| IBIS file stm32l552_562_wlcsp81_p.ibs
[IBIS ver]   4.2
[File name]  stm32l552_562_wlcsp81_p.ibs
[File Rev]   1.0
[Date]   04-10-2019
[Source]   Data Created at STMicroelectronics
[Notes]   File originated from ELDO simulations.
[Disclaimer] This information is for modeling purpose only and is
   not guaranted.
   The information is subject to change without notice.
[Copyright]  Copyright 2019 STMicroelectronics Inc.
|   Component stm32l552_562_wlcsp81_p
[Component] stm32l552_562_wlcsp81_p
[Manufacturer] STMicroelectronics
[Package]
| variable   typ   min   max
R_pkg  0  NA  NA
L_pkg  0  NA  NA
C_pkg  0  NA  NA
[Pin]   signal_name   model_name R_pin L_pin C_pin
A1 VDD POWER
A2 PC10 io8prog2m25m50m120m_sudq_ft
A3 PD2 io8prog2m25m50m120m_sudq_ft
A4 PG13 io8prog2m25m50m120m_sudq_i2c_ft
A5 VDDIO2 POWER
A6 PB5 io8prog2m25m50m120m_sudq_ft
A7 PB9 io8prog2m25m50m120m_sudq_i2c_ft
A8 VDD12_2 POWER
A9 VDD POWER
B1 VDDUSB POWER
B2 VSS GND
B3 PC12 io8prog2m25m50m120m_sudq_ft
B4 PG12 io8prog2m25m50m120m_sudq_ft
B5 VSS GND
B6 PB4 io8prog2m25m50m120m_sudq_i2c_ft
B7 PC13 io8prog2m25m50m120m_sudq_ft
B8 VSS GND
B9 VBAT POWER
C1 PA11 io8usblsfs_otg2
C2 PA12 io8usblsfs_otg2
C3 PC11 io8prog2m25m50m120m_sudq_ft
C4 PG10 io8prog2m25m50m120m_sudq_ft
C5 PG15 io8prog2m25m50m120m_sudq_ft
C6 PB6 io8prog2m25m50m120m_sudq_i2c_ft
C7 PB8 io8prog2m25m50m120m_sudq_i2c_ft
C8 PC15-OSC32_OUT io8prog2m25m50m120m_sudq_ft
C9 PC14-OSC32_IN io8prog2m25m50m120m_sudq_ft
D1 PA9 io8prog2m25m50m120m_sudq_ft
D2 PA13 io8prog2m25m50m120m_sudq_ft
D3 PA14 io8prog2m25m50m120m_sudq_i2c_ft
D4 PG9 io8prog2m25m50m120m_sudq_ft
D5 PG14 io8prog2m25m50m120m_sudq_i2c_ft
D6 PB7 io8prog2m25m50m120m_sudq_i2c_ft
D7 PH3-BOOT0 io8prog2m25m50m120m_sudq_ft
D8 PH1-OSC_OUT io8prog2m25m50m120m_sudq_ft
D9 PH0-OSC_IN io8prog2m25m50m120m_sudq_ft
E1 PC6 io8prog2m25m50m120m_sudq_ft
E2 PC7 io8prog2m25m50m120m_sudq_ft
E3 PA10 io8prog2m25m50m120m_sudq_ft
E4 PA15 io6usb_bmc_pd_cc_ft
E5 PG11 io8prog2m25m50m120m_sudq_ft
E6 PB3 io8prog2m25m50m120m_sudq_ft
E7 PC0 io8prog2m25m50m120m_sudq_i2c_ft
E8 VSS GND
E9 NRST ioreset_ft_v33
F1 PB15 io6usb_bmc_pd_cc_ft
F2 PB13 io8prog2m25m50m120m_sudq_i2c_ft
F3 PC8 io8prog2m25m50m120m_sudq_ft
F4 PA8 io8prog2m25m50m120m_sudq_i2c_ft
F5 PA3 io8prog2m25m50m120m_sudq_ft
F6 PA1 io8prog2m25m50m120m_sudq_ft
F7 PC2 io8prog2m25m50m120m_sudq_ft
F8 PC1 io8prog2m25m50m120m_sudq_i2c_ft
F9 VDD POWER
G1 PB14 io8prog2m25m50m120m_sudq_i2c_ft
G2 PB12 io8prog2m25m50m120m_sudq_ft
G3 PC9 io8prog2m25m50m120m_sudq_i2c_ft
G4 PC4 io8prog2m25m50m120m_sudq_ft
G5 PA6 io8prog2m25m50m120m_sudq_ft
G6 PA2 io8prog2m25m50m120m_sudq_ft
G7 PC3 io8prog2m25m50m120m_sudq_ft
G8 VREF+ POWER
G9 VSSA_VREF- GND
H1 VDD POWER
H2 VSS GND
H3 PE15 io8prog2m25m50m120m_sudq_ft
H4 PE14 io8prog2m25m50m120m_sudq_ft
H5 PB1 io8prog2m25m50m120m_sudq_ft
H6 PA5 io8prog2m25m50m120m_sudq_ft
H7 PA4 io8prog2m25m50m120m_sudq_ft
H8 PA0 io8prog2m25m50m120m_sudq_ft
H9 VDDA POWER
J1 VDD12_1 POWER
J2 PB11 io8prog2m25m50m120m_sudq_i2c_ft
J3 PB10 io8prog2m25m50m120m_sudq_i2c_ft
J4 PE13 io8prog2m25m50m120m_sudq_ft
J5 PB2 io8prog2m25m50m120m_sudq_ft
J6 PB0 io8prog2m25m50m120m_sudq_ft
J7 PA7 io8prog2m25m50m120m_sudq_i2c_ft
J8 VDD POWER
J9 VSS GND
[Model Selector] io6usb_bmc_pd_cc_ft
usb_bmc_emit_pdccpd  "BMC PD emitter  + PD"
usb_bmc_emit_pdcc3a0  "BMC PD emitter  + 3rd PU"
usb_bmc_emit_pdcc1a5  "BMC PD emitter  + 2nd PU"
usb_bmc_emit_pdccusb  "BMC PD emitter  + 1st PU"
usb_bmc_emit  "BMC PD emitter "
io2_pdcc_ft_3v3_lowspeed  "GPIO-3.3V range - low speed"
io2_pdcc_ft_3v3_mediumspeed  "GPIO-3.3V range - medium speed"
io2_pdcc_ft_3v3_lowspeed_pu  "GPIO-3.3V range - low speed - pull up"
io2_pdcc_ft_3v3_mediumspeed_pu  "GPIO-3.3V range - medium speed - pull up"
io2_pdcc_ft_3v3_lowspeed_pd  "GPIO-3.3V range - low speed - pull down"
io2_pdcc_ft_3v3_mediumspeed_pd  "GPIO-3.3V range - medium speed - pull down"
io2_pdcc_ft_1v8_lowspeed  "GPIO-1.8V range - low speed"
io2_pdcc_ft_1v8_mediumspeed  "GPIO-1.8V range - medium speed"
io2_pdcc_ft_1v8_lowspeed_pu  "GPIO-1.8V range - low speed - pull up"
io2_pdcc_ft_1v8_mediumspeed_pu  "GPIO-1.8V range - medium speed - pull up"
io2_pdcc_ft_1v8_lowspeed_pd  "GPIO-1.8V range - low speed - pull down"
io2_pdcc_ft_1v8_mediumspeed_pd  "GPIO-1.8V range - medium speed - pull down"
io2_pdcc_ft_1v2_lowspeed  "GPIO-1.2V range - low speed"
io2_pdcc_ft_1v2_mediumspeed  "GPIO-1.2V range - medium speed"
io2_pdcc_ft_1v2_lowspeed_pu  "GPIO-1.2V range - low speed - pull up"
io2_pdcc_ft_1v2_mediumspeed_pu  "GPIO-1.2V range - medium speed - pull up"
io2_pdcc_ft_1v2_lowspeed_pd  "GPIO-1.2V range - low speed - pull down"
io2_pdcc_ft_1v2_mediumspeed_pd  "GPIO-1.2V range - medium speed - pull down"
[Model Selector] io8prog2m25m50m120m_sudq_ft
iols8p_sudq_ft_pd_lv  "IO low speed, PD=40kOhm - 1P8V"
iols8p_sudq_ft_pu_lv  "IO low speed, PU=40kOhm - 1P8V"
iols8p_sudq_ft_lv  "IO low speed - 1P8V"
iols8p_sudq_ft_pd  "IO low speed, PD=40kOhm - 3P3V"
iols8p_sudq_ft_pu  "IO low speed, PU=40kOhm - 3P3V"
iols8p_sudq_ft  "IO low speed - 3P3V"
iofs8p_sudq_ft_pd_lv  "IO full speed, PD=40kOhm - 1P8V"
iofs8p_sudq_ft_pu_lv  "IO full speed, PU=40kOhm - 1P8V"
iofs8p_sudq_ft_lv  "IO full speed - 1P8V"
iofs8p_sudq_ft_pd  "IO full speed, PD=40kOhm - 3P3V"
iofs8p_sudq_ft_pu  "IO full speed, PU=40kOhm - 3P3V"
iofs8p_sudq_ft  "IO full speed - 3P3V"
ioms8p_sudq_ft_pd_lv  "IO medium speed, PD=40kOhm - 1P8V"
ioms8p_sudq_ft_pu_lv  "IO medium speed, PU=40kOhm - 1P8V"
ioms8p_sudq_ft_lv  "IO medium speed - 1P8V"
ioms8p_sudq_ft_pd  "IO medium speed, PD=40kOhm - 3P3V"
ioms8p_sudq_ft_pu  "IO medium speed, PU=40kOhm - 3P3V"
ioms8p_sudq_ft  "IO medium speed - 3P3V"
iohs8p_sudq_ft_pd_lv  "IO high speed, PD=40kOhm - 1P8V"
iohs8p_sudq_ft_pu_lv  "IO high speed, PU=40kOhm - 1P8V"
iohs8p_sudq_ft_lv  "IO high speed - 1P8V"
iohs8p_sudq_ft_pd  "IO high speed, PD=40kOhm - 3P3V"
iohs8p_sudq_ft_pu  "IO high speed, PU=40kOhm - 3P3V"
iohs8p_sudq_ft  "IO high speed - 3P3V"
[Model Selector] io8prog2m25m50m120m_sudq_i2c_ft
io8prog_1v8_i2c_pd  "5V Tol GPIO 1.8V range i2c functionality with pull down"
io8prog_1v8_i2c_pu  "5V Tol GPIO 1.8V range i2c functionality with pull up"
io8prog_1v8_i2c  "5V Tol GPIO 1.8V range i2c functionality"
io8prog_3v3_i2c_pd  "5V Tol GPIO 3.3V range i2c functionality with pull down"
io8prog_3v3_i2c_pu  "5V Tol GPIO 3.3V range i2c functionality with pull up"
io8prog_3v3_i2c  "5V Tol GPIO 3.3V range i2c functionality"
iols8p_sudq_ft_pd_lv  "IO low speed, PD=40kOhm - 1P8V"
iols8p_sudq_ft_pu_lv  "IO low speed, PU=40kOhm - 1P8V"
iols8p_sudq_ft_lv  "IO low speed - 1P8V"
iols8p_sudq_ft_pd  "IO low speed, PD=40kOhm - 3P3V"
iols8p_sudq_ft_pu  "IO low speed, PU=40kOhm - 3P3V"
iols8p_sudq_ft  "IO low speed - 3P3V"
iofs8p_sudq_ft_pd_lv  "IO full speed, PD=40kOhm - 1P8V"
iofs8p_sudq_ft_pu_lv  "IO full speed, PU=40kOhm - 1P8V"
iofs8p_sudq_ft_lv  "IO full speed - 1P8V"
iofs8p_sudq_ft_pd  "IO full speed, PD=40kOhm - 3P3V"
iofs8p_sudq_ft_pu  "IO full speed, PU=40kOhm - 3P3V"
iofs8p_sudq_ft  "IO full speed - 3P3V"
ioms8p_sudq_ft_pd_lv  "IO medium speed, PD=40kOhm - 1P8V"
ioms8p_sudq_ft_pu_lv  "IO medium speed, PU=40kOhm - 1P8V"
ioms8p_sudq_ft_lv  "IO medium speed - 1P8V"
ioms8p_sudq_ft_pd  "IO medium speed, PD=40kOhm - 3P3V"
ioms8p_sudq_ft_pu  "IO medium speed, PU=40kOhm - 3P3V"
ioms8p_sudq_ft  "IO medium speed - 3P3V"
iohs8p_sudq_ft_pd_lv  "IO high speed, PD=40kOhm - 1P8V"
iohs8p_sudq_ft_pu_lv  "IO high speed, PU=40kOhm - 1P8V"
iohs8p_sudq_ft_lv  "IO high speed - 1P8V"
iohs8p_sudq_ft_pd  "IO high speed, PD=40kOhm - 3P3V"
iohs8p_sudq_ft_pu  "IO high speed, PU=40kOhm - 3P3V"
iohs8p_sudq_ft  "IO high speed - 3P3V"
[Model Selector] io8usblsfs_otg2
usb_ls_pd  "USB Low Speed mode - Pull Down"
usb_ls_pu2  "USB Low Speed mode - Pull up 2"
usb_ls_pu  "USB Low Speed mode - Pull up"
usb_fs  "USB Low Speed mode"
usb_fs_pd  "USB Full Speed mode - Pull Down"
usb_fs_pu2  "USB Full Speed mode - Pull up 2"
usb_fs_pu  "USB Full Speed mode - Pull up"
[Model Selector] ioreset_ft_v33
ioreset_1v2_pu  "RESET 1.2V range with PU"
ioreset_1v2  "RESET 1.2V range"
ioreset_1v8_pu  "RESET 1.8V range with PU"
ioreset_1v8  "RESET 1.8V range"
ioreset_3v3_pu  "RESET 3.3V range with PU"
ioreset_3v3  "RESET 3.3V range"
| Models and submodels in the file (66): usb_bmc_emit_pdccpd (I/O), usb_bmc_emit_pdcc3a0 (I/O), usb_bmc_emit_pdcc1a5 (I/O), usb_bmc_emit_pdccusb (I/O), usb_bmc_emit (I/O), io2_pdcc_ft_3v3_lowspeed (I/O), io2_pdcc_ft_3v3_mediumspeed (I/O), io2_pdcc_ft_3v3_lowspeed_pu (I/O), io2_pdcc_ft_3v3_mediumspeed_pu (I/O), io2_pdcc_ft_3v3_lowspeed_pd (I/O), io2_pdcc_ft_3v3_mediumspeed_pd (I/O), io2_pdcc_ft_1v8_lowspeed (I/O), io2_pdcc_ft_1v8_mediumspeed (I/O), io2_pdcc_ft_1v8_lowspeed_pu (I/O), io2_pdcc_ft_1v8_mediumspeed_pu (I/O), io2_pdcc_ft_1v8_lowspeed_pd (I/O), io2_pdcc_ft_1v8_mediumspeed_pd (I/O), io2_pdcc_ft_1v2_lowspeed (I/O), io2_pdcc_ft_1v2_mediumspeed (I/O), io2_pdcc_ft_1v2_lowspeed_pu (I/O), io2_pdcc_ft_1v2_mediumspeed_pu (I/O), io2_pdcc_ft_1v2_lowspeed_pd (I/O), io2_pdcc_ft_1v2_mediumspeed_pd (I/O), iols8p_sudq_ft_pd_lv (I/O), iols8p_sudq_ft_pu_lv (I/O), iols8p_sudq_ft_lv (I/O), iols8p_sudq_ft_pd (I/O), iols8p_sudq_ft_pu (I/O), iols8p_sudq_ft (I/O), iofs8p_sudq_ft_pd_lv (I/O), iofs8p_sudq_ft_pu_lv (I/O), iofs8p_sudq_ft_lv (I/O), iofs8p_sudq_ft_pd (I/O), iofs8p_sudq_ft_pu (I/O), iofs8p_sudq_ft (I/O), ioms8p_sudq_ft_pd_lv (I/O), ioms8p_sudq_ft_pu_lv (I/O), ioms8p_sudq_ft_lv (I/O), ioms8p_sudq_ft_pd (I/O), ioms8p_sudq_ft_pu (I/O), ioms8p_sudq_ft (I/O), iohs8p_sudq_ft_pd_lv (I/O), iohs8p_sudq_ft_pu_lv (I/O), iohs8p_sudq_ft_lv (I/O), iohs8p_sudq_ft_pd (I/O), iohs8p_sudq_ft_pu (I/O), iohs8p_sudq_ft (I/O), io8prog_1v8_i2c_pd (I/O_open_drain), io8prog_1v8_i2c_pu (I/O_open_drain), io8prog_1v8_i2c (I/O_open_drain), io8prog_3v3_i2c_pd (I/O_open_drain), io8prog_3v3_i2c_pu (I/O_open_drain), io8prog_3v3_i2c (I/O_open_drain), usb_ls_pd (I/O), usb_ls_pu2 (I/O), usb_ls_pu (I/O), usb_fs (I/O), usb_fs_pd (I/O), usb_fs_pu2 (I/O), usb_fs_pu (I/O), ioreset_1v2_pu (I/O_open_drain), ioreset_1v2 (I/O_open_drain), ioreset_1v8_pu (I/O_open_drain), ioreset_1v8 (I/O_open_drain), ioreset_3v3_pu (I/O_open_drain), ioreset_3v3 (I/O_open_drain)
